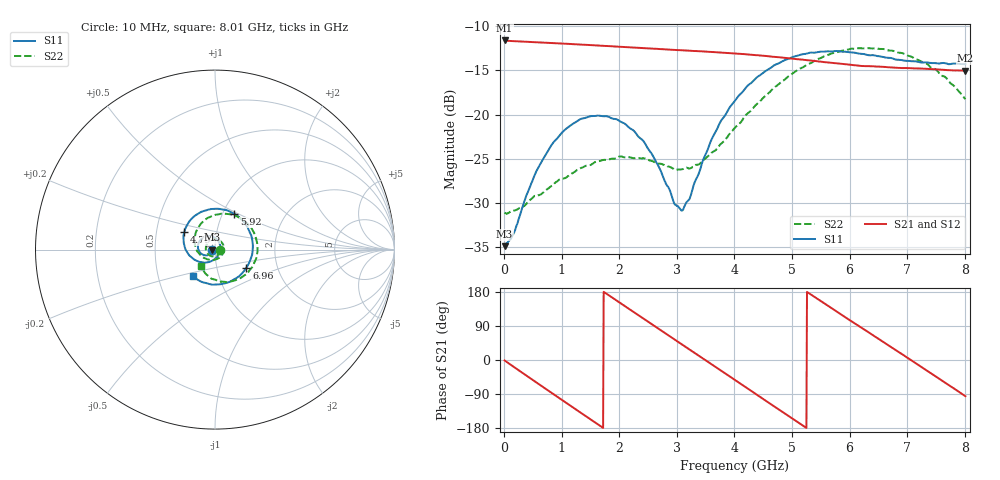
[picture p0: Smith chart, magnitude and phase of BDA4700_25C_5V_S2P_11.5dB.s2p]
!Agilent Technologies,E5071B,MY42404982,A.09.10
!Date: Mon Oct 20 13:31:51 2025
!Data & Calibration Information:
!Freq	S11:SOLT2(ON)	S21:SOLT2(ON)	S12:SOLT2(ON)	S22:SOLT2(ON)
# Hz S RI R 50
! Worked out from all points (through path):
!   801 points, 10 MHz to 8.01 GHz, reference 50 ohm
!   highest |S21| = -11.61 dB at 10 MHz (marker M1); lowest = -15.0 dB at 8.01 GHz (marker M2)
!   group delay of S21, straight-line fit = 282 ps
!   lowest |S11| = -34.9 dB at 10 MHz (marker M3), VSWR 1.04, Z = 48.2 - j0.104 ohm
!   |S11| at or under -10 dB: start of sweep to end of sweep
!   |S22| runs from -31.2 to -12.5 dB; largest |S21 - S12| = 0.002
!   S11 on the Smith chart (normalised r, x): 10 MHz: 0.96, -0.00; 4.79 GHz: 0.70, +0.14; 5.92 GHz: 1.14, +0.48; 6.96 GHz: 1.39, -0.29; 8.01 GHz: 0.75, -0.23
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1e7  -0.0179 -0.00108  0.2626 -0.00573  0.2625 -0.00603  0.0279 -0.00147
1.6e8  -0.0188 -0.00934  0.2488 -0.0769  0.2487 -0.077  0.027 -0.0093
5.1e8  -0.0336 -0.0279  0.1516 -0.2076  0.1516 -0.2077  0.0142 -0.0311
7.2e8  -0.0496 -0.0321  0.0627 -0.2471  0.0629 -0.2471  -0.0018 -0.0371
1.02e9  -0.0765 -0.023  -0.073 -0.2413  -0.0731 -0.2413  -0.0283 -0.0329
1.35e9  -0.0946 0.00611  -0.1933 -0.1566  -0.1933 -0.1567  -0.0496 -0.00628
1.94e9  -0.0664 0.0669  -0.2255 0.0899  -0.2255 0.09  -0.0251 0.0505
2.41e9  -0.00874 0.0709  -0.0819 0.223  -0.0819 0.2232  0.0273 0.0497
2.68e9  0.0181 0.0477  0.03 0.2333  0.03 0.2332  0.0469 0.024
2.96e9  0.0294 0.0104  0.1358 0.1883  0.1359 0.1881  0.0483 -0.00861
3.1e9  0.027 -0.00959  0.1774 0.1478  0.1769 0.1484  0.042 -0.0256
3.54e9  -0.0158 -0.0619  0.226 -0.0192  0.226 -0.0195  -0.00679 -0.0577
4.01e9  -0.1026 -0.0619  0.1341 -0.1768  0.1342 -0.1766  -0.0759 -0.0362
4.39e9  -0.1625 -0.00264  -0.00641 -0.2165  -0.00636 -0.2171  -0.112 0.0255
4.79e9  -0.1708 0.0975  -0.1428 -0.155  -0.1422 -0.1558  -0.0993 0.1133
5.35e9  -0.0674 0.2137  -0.199 0.0331  -0.1991 0.0326  0.0197 0.1963
5.92e9  0.1082 0.1995  -0.076 0.1772  -0.0765 0.177  0.1787 0.1462
6.3e9  0.1882 0.1093  0.0451 0.1824  0.0461 0.1816  0.234 0.0403
6.68e9  0.2088 -0.0156  0.1457 0.114  0.1462 0.114  0.2186 -0.0744
6.96e9  0.1749 -0.1002  0.1803 0.0332  0.1803 0.0323  0.1682 -0.1404
7.49e9  0.0316 -0.193  0.132 -0.123  0.1318 -0.1232  0.0235 -0.1792
8.01e9  -0.124 -0.1484  -0.0171 -0.1762  -0.0169 -0.1764  -0.0784 -0.0937
